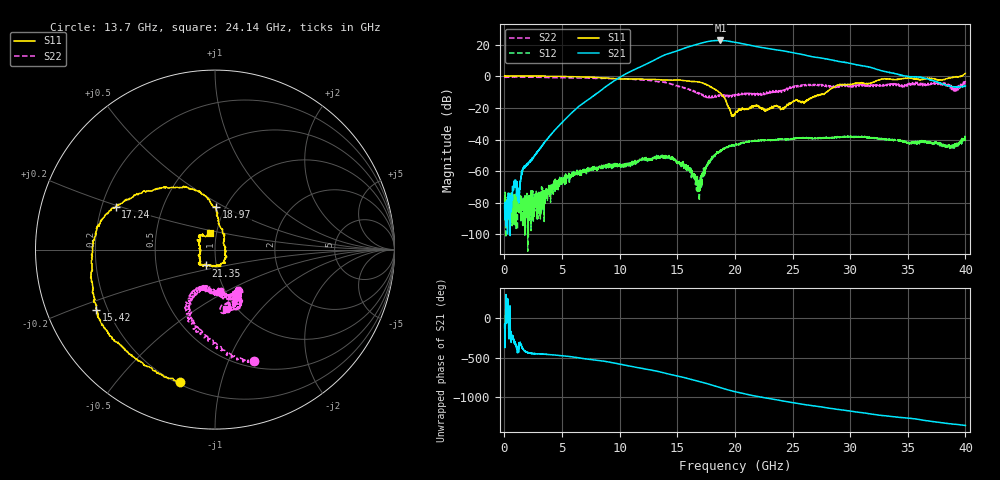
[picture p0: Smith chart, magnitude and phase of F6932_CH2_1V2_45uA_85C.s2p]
!Keysight Technologies,M9807A,MY58100526,A.15.20.05
!Date: Tuesday, August 01, 2023 10:54:57
!Correction: S11(Cdelta 2-Port  )
!S21(Cdelta 2-Port  )
!S12(Cdelta 2-Port  )
!S22(Cdelta 2-Port  )
!S2P File: Measurements: S11, S21, S12, S22:
# Hz S  dB  R 50
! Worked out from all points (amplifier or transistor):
!   4000 points, 10 MHz to 40 GHz, reference 50 ohm
!   highest |S21| = 22.6 dB at 18.74 GHz (marker M1)
!   |S21| within 3 dB of that: 16.45 GHz to 21.3 GHz (4.849 GHz wide, 25.7 % of centre)
!   unconditionally stable (mu >= 1): 3.64 GHz to 3.69 GHz; 3.77 GHz to 3.82 GHz; 3.9 GHz to 39.62 GHz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
!   at 6.67 GHz: K = 120.30, MAG = -1.5 dB, |S12| = -62.5 dB
!   at 20.01 GHz: K = 5.85, MAG = 21.7 dB, |S12| = -43.3 dB
!   at 40 GHz: K = -31.32, MSG = 17.1 dB, |S12| = -40.4 dB
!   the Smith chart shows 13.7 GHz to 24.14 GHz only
!   S11 on the Smith chart (normalised r, x): 13.7 GHz: 0.21, -0.75; 15.42 GHz: 0.16, -0.23; 17.24 GHz: 0.26, +0.19; 18.97 GHz: 0.90, +0.46; 21.35 GHz: 0.89, -0.16; 24.14 GHz: 0.93, +0.18
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1e7  0.13 178.6  -82.00 -120.2  -77.17 -148.3  -0.82 178.3
6.68e9  -0.46 66.9  -17.88 -148.1  -60.73 142.7  -1.09 60.8
1.089e10  -1.72 -38.8  2.82 112.4  -56.23 92.0  -1.78 -16.1
1.334e10  -2.21 -92.9  11.46 44.3  -51.25 49.4  -3.51 -62.1
1.37e10  -2.33 -104.6  12.75 31.9  -51.18 47.5  -3.61 -70.9
1.542e10  -2.61 -153.1  17.16 -26.9  -55.40 -4.9  -6.95 -105.5
1.633e10  -3.32 179.8  19.33 -60.1  -62.18 -25.3  -9.39 -116.2
1.724e10  -4.40 156.6  21.21 -95.0  -62.49 159.9  -12.14 -109.9
1.793e10  -6.84 130.7  22.24 -125.1  -52.23 132.0  -13.36 -100.1
1.874e10  -10.86 97.5  22.60 -161.1  -46.53 96.2  -12.47 -83.3
1.897e10  -12.46 88.5  22.53 -171.0  -45.99 89.2  -11.80 -82.9
1.943e10  -19.44 66.6  22.16 169.8  -44.34 71.4  -13.21 -80.0
2.001e10  -23.84 -29.7  21.45 147.7  -43.32 52.5  -12.33 -85.0
2.066e10  -20.55 -70.4  20.55 125.4  -41.83 38.3  -11.63 -71.3
2.135e10  -19.85 -120.0  19.53 104.4  -40.98 19.1  -11.81 -64.0
2.27e10  -21.33 180.0  17.69 67.9  -40.28 -8.9  -11.20 -67.0
2.414e10  -20.07 106.5  16.10 31.2  -39.99 -33.5  -9.48 -79.4
2.667e10  -13.70 2.4  12.36 -28.8  -39.24 -78.8  -5.13 -96.1
2.827e10  -8.24 -48.6  10.45 -63.5  -38.73 -101.4  -6.10 -105.2
3.025e10  -4.99 -77.4  7.71 -104.1  -38.40 -136.2  -6.71 -128.5
3.334e10  -1.76 -128.8  2.49 -163.1  -40.07 173.2  -5.79 -160.4
4e10  1.77 109.8  -6.25 79.3  -40.37 38.7  -3.83 112.4
